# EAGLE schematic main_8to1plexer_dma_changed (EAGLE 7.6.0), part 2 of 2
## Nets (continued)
ZBUS0: IC6.3(1D) IC7.3(1D) IC48.3(1D) IC96.2(1A) IC97.2(1A) IC144.14(D1) IC175.4(B:I0) IC184.3(1D) IC189.3(1D) IC197.1(A:I0) IC216.3(1D) IC241.3(1C3) IC248.14(D1) RN5.1
ZBUS1: IC96.5(2A) IC97.5(2A) IC144.13(D2) IC175.5(B:I1) IC184.4(2D) IC197.2(A:I1) IC216.4(2D) IC243.3(1C3) IC248.13(D2) RN5.2
ZBUS2: IC96.11(3A) IC97.11(3A) IC144.12(D3) IC177.5(B:I1) IC184.7(3D) IC197.3(A:I2) IC216.7(3D) IC248.12(D3) IC255.3(1C3) RN5.3
ZBUS3: IC96.14(4A) IC97.14(4A) IC144.11(D4) IC184.8(4D) IC192.5(B:I1) IC197.12(A:I3) IC216.8(4D) IC248.11(D4) IC256.3(1C3) RN5.4
ZBUS4: IC94.2(1A) IC95.2(1A) IC128.14(D1) IC184.13(5D) IC193.5(B:I1) IC197.13(A:I4) IC208.3(1C3) IC216.13(5D) IC249.14(D1) RN5.5
ZBUS5: IC94.5(2A) IC95.5(2A) IC128.13(D2) IC184.14(6D) IC194.5(B:I1) IC199.2(A:I1) IC216.14(6D) IC249.13(D2) RN5.6
ZBUS6: IC94.11(3A) IC95.11(3A) IC128.12(D3) IC184.17(7D) IC199.3(A:I2) IC200.5(B:I1) IC216.17(7D) IC249.12(D3) RN5.7
ZBUS7: IC6.18(8D) IC7.18(8D) IC48.18(8D) IC80.5(B:I1) IC94.14(4A) IC95.14(4A) IC128.11(D4) IC184.18(8D) IC189.18(8D) IC199.12(A:I3) IC209.5(B:I1) IC216.18(8D) IC249.11(D4) IC255.5(1C1) RN5.8
ZF: IC120.2(A:I1) IC122.2(A1) IC155.6(1C0) IC227.2(Q1) IC241.6(1C0)
ZF_FROM_ALU: IC120.1(A:I0) IC121.2(1A) IC124.1(A:I0) IC127.1(A:I0) IC155.4(1C2) IC199.5(A:O) IC241.5(1C1)
ZF_IN_SRC_0: IC241.14(A)
ZF_IN_SRC_1: IC241.2(B)
~CLK: IC32.11(CLK) IC33.11(CLK)
~RST: IC32.1(CLR) IC33.1(CLR) IC44.4(A:PRE) IC54.4(B:O) IC162.1(CLR) IC195.1(A:I0) IC204.1(A:CLR) IC207.2(A:I1) IC218.1(A:I0) IC219.1(A:I0) IC220.2(A:I1) IC223.2(A:I1) IC224.2(A:I1) IC225.2(A:I1) IC227.1(CLR)
Unconnected: IC1.11(CLK) IC1.18(8D) IC2.12(Y7) IC2.13(Y6) IC2.14(Y5) IC3.12(Y7) IC3.13(Y6) IC3.14(Y5) IC4.11(CLK) IC5.11(CLK) IC6.4(2D) IC6.7(3D) IC6.8(4D) IC6.11(CLK) IC6.13(5D) IC6.14(6D) IC6.17(7D) IC7.4(2D) IC7.7(3D) IC7.8(4D) IC7.13(5D) IC7.14(6D) IC7.17(7D) IC8.6(A:!Q) IC8.8(B:!Q) IC8.9(B:Q) IC8.10(B:PRE) IC8.11(B:CLK) IC8.12(B:D) IC8.13(B:CLR) IC9.12(Y7) IC9.13(Y6) IC9.14(Y5) IC10.3(B:Y4) IC10.5(B:Y3) IC10.7(B:Y2) IC10.9(B:Y1) IC10.11(B:A1) IC10.13(B:A2) IC10.15(B:A3) IC10.17(B:A4) IC10.19(B:G) IC11.3(B:Y4) IC11.5(B:Y3) IC11.7(B:Y2) IC11.9(B:Y1) IC11.11(B:A1) IC11.13(B:A2) IC11.15(B:A3) IC11.17(B:A4) IC11.19(B:G) IC12.3(B:Y4) IC12.5(B:Y3) IC12.7(B:Y2) IC12.9(B:Y1) IC12.11(B:A1) IC12.13(B:A2) IC12.15(B:A3) IC12.17(B:A4) IC12.19(B:G) IC13.3(B:Y4) IC13.5(B:Y3) IC13.7(B:Y2) IC13.9(B:Y1) IC13.11(B:A1) IC13.13(B:A2) IC13.15(B:A3) IC13.17(B:A4) IC13.19(B:G) IC14.14(A=B) IC14.15(P) IC14.17(G) IC15.14(A=B) IC15.15(P) IC15.17(G) IC16.11(CLK) IC17.11(CLK) IC18.1(A:I0) IC18.2(A:I1) IC18.3(A:O) IC18.8(C:O) IC18.9(C:I0) IC18.10(C:I1) IC18.11(D:O) IC18.12(D:I0) IC18.13(D:I1) IC19.2(A1) IC19.3(A2) IC19.4(A3) IC19.5(A4) IC19.6(A5) IC19.7(A6) IC19.8(A7) IC19.9(A8) IC19.12(Y7) IC19.13(Y6) IC19.19(G2) IC20.1(D3) IC20.2(D2) IC20.3(D1) IC20.4(D0) IC20.6(W) IC20.7(G) IC20.9(C) IC20.10(B) IC20.11(A) IC20.12(D7) IC20.13(D6) IC20.14(D5) IC20.15(D4) IC21.11(CLK) IC24.1(A:G) IC24.2(A:A1) IC24.4(A:A2) IC24.6(A:A3) IC24.8(A:A4) IC24.12(A:Y4) IC24.14(A:Y3) IC24.16(A:Y2) IC24.18(A:Y1) IC25.1(A:G) IC25.2(A:A1) IC25.4(A:A2) IC25.6(A:A3) IC25.8(A:A4) IC25.12(A:Y4) IC25.14(A:Y3) IC25.16(A:Y2) IC25.18(A:Y1) IC26.1(A:G) IC26.2(A:A1) IC26.4(A:A2) IC26.6(A:A3) IC26.8(A:A4) IC26.12(A:Y4) IC26.14(A:Y3) IC26.16(A:Y2) IC26.18(A:Y1) IC27.1(A:G) IC27.2(A:A1) IC27.4(A:A2) IC27.6(A:A3) IC27.8(A:A4) IC27.12(A:Y4) IC27.14(A:Y3) IC27.16(A:Y2) IC27.18(A:Y1) IC28.12(Y7) IC28.13(Y6) IC28.14(Y5) IC29.12(Y7) IC29.13(Y6) IC29.14(Y5) IC30.3(B:Y4) IC30.5(B:Y3) IC30.7(B:Y2) IC30.9(B:Y1) IC30.11(B:A1) IC30.13(B:A2) IC30.15(B:A3) IC30.17(B:A4) IC30.19(B:G) IC31.3(B:Y4) IC31.5(B:Y3) IC31.7(B:Y2) IC31.9(B:Y1) IC31.11(B:A1) IC31.13(B:A2) IC31.15(B:A3) IC31.17(B:A4) IC31.19(B:G) IC34.6(W) IC34.7(G) IC34.9(C) IC34.10(B) IC34.11(A) IC34.12(D7) IC34.13(D6) IC35.6(W) IC35.7(G) IC35.9(C) IC35.10(B) IC35.11(A) IC35.12(D7) IC35.13(D6) IC36.6(W) IC36.7(G) IC36.9(C) IC36.10(B) IC36.11(A) IC36.12(D7) IC36.13(D6) IC37.6(W) IC37.7(G) IC37.9(C) IC37.10(B) IC37.11(A) IC37.12(D7) IC37.13(D6) IC38.6(W) IC38.7(G) IC38.9(C) IC38.10(B) IC38.11(A) IC38.12(D7) IC38.13(D6) IC39.4(B:I0) IC39.5(B:I1) IC39.6(B:O) IC39.8(C:O) IC39.9(C:I0) IC39.10(C:I1) IC39.11(D:O) IC39.12(D:I0) IC39.13(D:I1) IC40.6(W) IC40.7(G) IC40.9(C) IC40.10(B) IC40.11(A) IC40.12(D7) IC40.13(D6) IC41.6(W) IC41.7(G) IC41.9(C) IC41.10(B) IC41.11(A) IC41.12(D7) IC41.13(D6) IC42.4(B:I0) IC42.5(B:I1) IC42.6(B:O) IC42.8(C:O) IC42.9(C:I0) IC42.10(C:I1) IC42.11(D:O) IC42.12(D:I0) IC42.13(D:I1) IC43.1(A:I) IC43.2(A:O) IC43.5(C:I) IC43.6(C:O) IC43.8(D:O) IC43.9(D:I) IC43.10(E:O) IC43.11(E:I) IC43.12(F:O) IC43.13(F:I) IC44.6(A:!Q) IC44.8(B:!Q) IC44.9(B:Q) IC44.10(B:PRE) IC44.11(B:CLK) IC44.12(B:D) IC44.13(B:CLR) IC45.4(B:I0) IC45.5(B:I1) IC45.6(B:O) IC45.8(C:O) IC45.9(C:I0) IC45.10(C:I1) IC45.11(D:O) IC45.12(D:I0) IC45.13(D:I1) IC46.1(A:I0) IC46.2(A:I1) IC46.3(A:O) IC46.8(C:O) IC46.9(C:I0) IC46.10(C:I1) IC46.11(D:O) IC46.12(D:I0) IC46.13(D:I1) IC47.4(B:I0) IC47.5(B:I1) IC47.6(B:O) IC47.8(C:O) IC47.9(C:I0) IC47.10(C:I1) IC47.11(D:O) IC47.12(D:I0) IC47.13(D:I1) IC48.4(2D) IC48.7(3D) IC48.8(4D) IC48.11(CLK) IC48.13(5D) IC48.14(6D) IC48.17(7D) IC50.1(S2) IC50.10(S4) IC50.13(S3) IC51.1(S2) IC51.4(S1) IC51.10(S4) IC51.13(S3) IC52.1(S2) IC52.4(S1) IC52.10(S4) IC52.13(S3) IC53.4(S1) IC53.9(C4) IC53.10(S4) IC53.13(S3) IC54.1(A:I) IC54.2(A:O) IC54.5(C:I) IC54.6(C:O) IC54.8(D:O) IC54.9(D:I) IC54.10(E:O) IC54.11(E:I) IC54.12(F:O) IC54.13(F:I) IC56.9(2Y) IC56.10(2C0) IC56.11(2C1) IC56.12(2C2) IC56.13(2C3) IC57.5(C:I) IC57.6(C:O) IC57.8(D:O) IC57.9(D:I) IC57.10(E:O) IC57.11(E:I) IC57.12(F:O) IC57.13(F:I) IC58.4(B:I0) IC58.5(B:I1) IC58.6(B:O) IC58.8(C:O) IC58.9(C:I0) IC58.10(C:I1) IC58.11(D:O) IC58.12(D:I0) IC58.13(D:I1) IC59.3(B:I) IC59.4(B:O) IC59.5(C:I) IC59.6(C:O) IC59.8(D:O) IC59.9(D:I) IC59.10(E:O) IC59.11(E:I) IC59.12(F:O) IC59.13(F:I) IC60.1(CLR) IC60.9(Q4) IC60.12(Q5) IC60.15(Q6) IC60.16(Q7) IC60.19(Q8) IC61.1(CLR) IC61.2(Q1) IC61.5(Q2) IC61.6(Q3) IC61.9(Q4) IC61.12(Q5) IC61.15(Q6) IC61.16(Q7) IC61.19(Q8) IC62.1(CLR) IC62.2(Q1) IC62.5(Q2) IC62.6(Q3) IC62.9(Q4) IC62.12(Q5) IC62.15(Q6) IC62.16(Q7) IC62.19(Q8) IC64.3(B:I0) IC64.4(B:I1) IC64.5(B:I2) IC64.6(B:O) IC64.8(C:O) IC64.9(C:I0) IC64.10(C:I1) IC64.11(C:I2) IC65.4(B:O) IC65.5(B:I0) IC65.6(B:I1) IC65.8(C:I0) IC65.9(C:I1) IC65.10(C:O) IC65.11(D:I0) IC65.12(D:I1) IC65.13(D:O) IC66.4(B:O) IC66.5(B:I0) IC66.6(B:I1) IC66.8(C:I0) IC66.9(C:I1) IC66.10(C:O) IC66.11(D:I0) IC66.12(D:I1) IC66.13(D:O) IC67.1(A:I0) IC67.2(A:I1) IC67.3(A:O) IC67.8(C:O) IC67.9(C:I0) IC67.10(C:I1) IC67.11(D:O) IC67.12(D:I0) IC67.13(D:I1) IC68.9(3Y) IC68.12(4Y) IC69.1(A:G) IC69.2(A:A1) IC69.3(B:Y4) IC69.4(A:A2) IC69.6(A:A3) IC69.8(A:A4) IC69.12(A:Y4) IC69.14(A:Y3) IC69.16(A:Y2) IC69.18(A:Y1) IC70.6(W) IC71.6(W) IC71.7(G) IC71.9(C) IC71.10(B) IC71.11(A) IC71.12(D7) IC71.13(D6) IC72.1(A:I0) IC72.2(A:I1) IC72.3(A:O) IC72.8(C:O) IC72.9(C:I0) IC72.10(C:I1) IC72.11(D:O) IC72.12(D:I0) IC72.13(D:I1) IC73.6(W) IC73.7(G) IC73.9(C) IC73.10(B) IC73.11(A) IC73.12(D7) IC73.13(D6) IC74.1(A:I0) IC74.2(A:I1) IC74.3(A:O) IC74.8(C:O) IC74.9(C:I0) IC74.10(C:I1) IC74.11(D:O) IC74.12(D:I0) IC74.13(D:I1) IC75.2(Q1) IC75.5(Q2) IC75.6(Q3) IC75.9(Q4) IC75.12(Q5) IC75.15(Q6) IC75.16(Q7) IC75.19(Q8) IC76.2(Q1) IC77.2(Q1) IC78.2(Q1) IC78.5(Q2) IC78.6(Q3) IC78.9(Q4) IC78.12(Q5) IC78.15(Q6) IC78.16(Q7) IC78.19(Q8) IC79.2(Q1) IC79.5(Q2) IC79.6(Q3) IC79.9(Q4) IC79.12(Q5) IC79.15(Q6) IC79.16(Q7) IC79.19(Q8) IC80.1(A:I0) IC80.2(A:I1) IC80.3(A:O) IC80.8(C:O) IC80.9(C:I0) IC80.10(C:I1) IC80.11(D:O) IC80.12(D:I0) IC80.13(D:I1) IC81.1(A:I0) IC81.2(A:I1) IC81.3(A:O) IC81.8(C:O) IC81.9(C:I0) IC81.10(C:I1) IC81.11(D:O) IC81.12(D:I0) IC81.13(D:I1) IC82.11(CLK) IC83.1(A:I) IC83.2(A:O) IC83.5(C:I) IC83.6(C:O) IC83.8(D:O) IC83.9(D:I) IC83.10(E:O) IC83.11(E:I) IC83.12(F:O) IC83.13(F:I) IC84.1(A:I) IC84.2(A:O) IC84.5(C:I) IC84.6(C:O) IC84.8(D:O) IC84.9(D:I) IC84.10(E:O) IC84.11(E:I) IC84.12(F:O) IC84.13(F:I) IC85.3(B:I0) IC85.4(B:I1) IC85.5(B:I2) IC85.6(B:O) IC85.8(C:O) IC85.9(C:I0) IC85.10(C:I1) IC85.11(C:I2) IC86.11(CLK) IC87.2(A:S1) IC87.5(C:R) IC87.6(C:S) IC87.7(C:Q) IC87.9(B:Q) IC87.10(B:R) IC87.11(B:S1) IC87.12(B:S2) IC87.13(D:Q) IC87.14(D:R) IC87.15(D:S) IC88.11(CLK) IC89.3(B:Y4) IC89.5(B:Y3) IC89.7(B:Y2) IC89.9(B:Y1) IC89.11(B:A1) IC89.13(B:A2) IC89.15(B:A3) IC89.17(B:A4) IC89.19(B:G) IC90.3(B:Y4) IC90.5(B:Y3) IC90.7(B:Y2) IC90.9(B:Y1) IC90.11(B:A1) IC90.13(B:A2) IC90.15(B:A3) IC90.17(B:A4) IC90.19(B:G) IC91.3(B:Y4) IC91.5(B:Y3) IC91.7(B:Y2) IC91.9(B:Y1) IC91.11(B:A1) IC91.13(B:A2) IC91.15(B:A3) IC91.17(B:A4) IC91.19(B:G) IC92.3(B:Y4) IC92.5(B:Y3) IC92.7(B:Y2) IC92.9(B:Y1) IC92.11(B:A1) IC92.13(B:A2) IC92.15(B:A3) IC92.17(B:A4) IC92.19(B:G) IC93.11(CLK) IC98.11(CLK) IC99.11(CLK) IC100.11(CLK) IC101.11(CLK) IC102.12(Y7) IC102.13(Y6) IC102.14(Y5) IC103.12(Y7) IC103.13(Y6) IC103.14(Y5) IC103.15(Y4) IC103.16(Y3) IC103.17(Y2) IC104.12(Y7) IC104.13(Y6) IC104.14(Y5) IC104.15(Y4) IC104.16(Y3) IC104.17(Y2) IC105.1(A:G) IC105.2(A:A1) IC105.4(A:A2) IC105.6(A:A3) IC105.8(A:A4) IC105.12(A:Y4) IC105.14(A:Y3) IC105.16(A:Y2) IC105.18(A:Y1) IC106.1(A:G) IC106.2(A:A1) IC106.4(A:A2) IC106.6(A:A3) IC106.8(A:A4) IC106.12(A:Y4) IC106.14(A:Y3) IC106.16(A:Y2) IC106.18(A:Y1) IC107.1(A:G) IC107.2(A:A1) IC107.4(A:A2) IC107.6(A:A3) IC107.8(A:A4) IC107.12(A:Y4) IC107.14(A:Y3) IC107.16(A:Y2) IC107.18(A:Y1) IC108.1(A:G) IC108.2(A:A1) IC108.4(A:A2) IC108.6(A:A3) IC108.8(A:A4) IC108.12(A:Y4) IC108.14(A:Y3) IC108.16(A:Y2) IC108.18(A:Y1) IC109.1(A:G) IC109.2(A:A1) IC109.4(A:A2) IC109.6(A:A3) IC109.8(A:A4) IC109.12(A:Y4) IC109.14(A:Y3) IC109.16(A:Y2) IC109.18(A:Y1) IC110.1(A:G) IC110.2(A:A1) IC110.4(A:A2) IC110.6(A:A3) IC110.8(A:A4) IC110.12(A:Y4) IC110.14(A:Y3) IC110.16(A:Y2) IC110.18(A:Y1) IC111.1(A:G) IC111.2(A:A1) IC111.4(A:A2) IC111.6(A:A3) IC111.8(A:A4) IC111.12(A:Y4) IC111.14(A:Y3) IC111.16(A:Y2) IC111.18(A:Y1) IC112.1(A:G) IC112.2(A:A1) IC112.4(A:A2) IC112.6(A:A3) IC112.8(A:A4) IC112.12(A:Y4) IC112.14(A:Y3) IC112.16(A:Y2) IC112.18(A:Y1) IC113.13(Y6) IC113.14(Y5) IC113.19(G2) IC114.13(Y6) IC114.14(Y5) IC114.19(G2) IC115.13(Y6) IC115.14(Y5) IC117.12(Y7) IC117.13(Y6) IC117.14(Y5) IC118.6(3Q) IC118.7(3D) IC118.8(4D) IC118.9(4Q) IC118.11(CLK) IC118.12(5Q) IC118.13(5D) IC118.14(6D) IC118.15(6Q) IC118.16(7Q) IC118.17(7D) IC118.18(8D) IC118.19(8Q) IC119.1(A:I) IC119.2(A:O) IC119.5(C:I) IC119.6(C:O) IC119.8(D:O) IC119.9(D:I) IC119.10(E:O) IC119.11(E:I) IC119.12(F:O) IC119.13(F:I) IC120.4(B:I0) IC120.5(B:I1) IC120.6(B:O) IC120.8(C:O) IC120.9(C:I0) IC120.10(C:I1) IC120.11(D:O) IC120.12(D:I0) IC120.13(D:I1) IC121.4(1Y) IC121.5(2A) IC121.6(2B) IC121.7(2Y) IC121.9(3Y) IC121.10(3B) IC121.11(3A) IC121.12(4Y) IC121.13(4B) IC121.14(4A) IC122.12(Y7) IC122.13(Y6) IC122.14(Y5) IC123.11(CLK) IC123.18(8D) IC124.4(B:I0) IC124.5(B:I1) IC124.6(B:O) IC124.8(C:O) IC124.9(C:I0) IC124.10(C:I1) IC124.11(D:O) IC124.12(D:I0) IC124.13(D:I1) IC126.11(CLK) IC126.12(5Q) IC126.13(5D) IC126.14(6D) IC126.15(6Q) IC126.16(7Q) IC126.17(7D) IC126.18(8D) IC126.19(8Q) IC127.4(B:I0) IC127.5(B:I1) IC127.6(B:O) IC127.8(C:O) IC127.9(C:I0) IC127.10(C:I1) IC127.11(D:O) IC127.12(D:I0) IC127.13(D:I1) IC129.6(W) IC129.7(G) IC129.9(C) IC129.10(B) IC129.11(A) IC129.12(D7) IC129.13(D6) IC130.1(A:I0) IC130.2(A:I1) IC130.3(A:O) IC130.8(C:O) IC130.9(C:I0) IC130.10(C:I1) IC130.11(D:O) IC130.12(D:I0) IC130.13(D:I1) IC131.4(B:O) IC131.5(B:I0) IC131.6(B:I1) IC131.8(C:I0) IC131.9(C:I1) IC131.10(C:O) IC131.11(D:I0) IC131.12(D:I1) IC131.13(D:O) IC132.3(B:I0) IC132.4(B:I1) IC132.5(B:I2) IC132.6(B:O) IC132.8(C:O) IC132.9(C:I0) IC132.10(C:I1) IC132.11(C:I2) IC133.3(A:O) IC133.4(B:I0) IC133.5(B:I1) IC133.6(B:O) IC133.8(C:O) IC133.9(C:I0) IC133.10(C:I1) IC133.11(D:O) IC133.12(D:I0) IC133.13(D:I1) IC134.2(Q1) IC134.5(Q2) IC134.6(Q3) IC134.9(Q4) IC134.12(Q5) IC134.15(Q6) IC134.16(Q7) IC134.19(Q8) IC135.2(Q1) IC135.5(Q2) IC135.6(Q3) IC135.9(Q4) IC135.12(Q5) IC135.15(Q6) IC135.16(Q7) IC135.19(Q8) IC136.2(Q1) IC136.5(Q2) IC136.6(Q3) IC136.9(Q4) IC136.12(Q5) IC136.15(Q6) IC136.16(Q7) IC136.19(Q8) IC137.2(Q1) IC137.5(Q2) IC137.6(Q3) IC137.9(Q4) IC137.12(Q5) IC137.15(Q6) IC137.16(Q7) IC137.19(Q8) IC138.3(B:I0) IC138.4(B:I1) IC138.5(B:I2) IC138.6(B:O) IC138.8(C:O) IC138.9(C:I0) IC138.10(C:I1) IC138.11(C:I2) IC139.4(Q2) IC139.5(Q3) IC139.6(Q4) IC139.11(D4) IC139.12(D3) IC139.13(D2) IC140.12(Y7) IC140.13(Y6) IC140.14(Y5) IC140.15(Y4) IC140.16(Y3) IC140.17(Y2) IC141.3(B:I0) IC141.4(B:I1) IC141.5(B:I2) IC141.6(B:O) IC141.8(C:O) IC141.9(C:I0) IC141.10(C:I1) IC141.11(C:I2) IC142.6(W) IC142.7(G) IC142.9(C) IC142.10(B) IC142.11(A) IC142.12(D7) IC142.13(D6) IC143.4(B:I0) IC143.5(B:I1) IC143.6(B:O) IC143.8(C:O) IC143.9(C:I0) IC143.10(C:I1) IC143.11(D:O) IC143.12(D:I0) IC143.13(D:I1) IC145.12(Y7) IC145.13(Y6) IC145.14(Y5) IC146.12(Y7) IC146.13(Y6) IC146.14(Y5) IC147.1(A:I0) IC147.2(A:I1) IC147.3(A:O) IC147.8(C:O) IC147.9(C:I0) IC147.10(C:I1) IC147.11(D:O) IC147.12(D:I0) IC147.13(D:I1) IC148.4(B:I0) IC148.5(B:I1) IC148.6(B:O) IC148.8(C:O) IC148.9(C:I0) IC148.10(C:I1) IC148.11(D:O) IC148.12(D:I0) IC148.13(D:I1) IC149.1(A:I) IC149.2(A:O) IC149.5(C:I) IC149.6(C:O) IC149.8(D:O) IC149.9(D:I) IC149.10(E:O) IC149.11(E:I) IC149.12(F:O) IC149.13(F:I) IC150.3(B:I0) IC150.4(B:I1) IC150.5(B:I2) IC150.6(B:O) IC150.8(C:O) IC150.9(C:I0) IC150.10(C:I1) IC150.11(C:I2) IC151.3(B:I0) IC151.4(B:I1) IC151.5(B:I2) IC151.6(B:O) IC151.8(C:O) IC151.9(C:I0) IC151.10(C:I1) IC151.11(C:I2) IC152.1(A:I0) IC152.2(A:I1) IC152.3(A:O) IC152.4(B:I0) IC152.5(B:I1) IC152.6(B:O) IC152.11(D:O) IC152.12(D:I0) IC152.13(D:I1) IC153.11(CLK) IC155.3(1C3) IC155.13(2C3) IC156.3(1C3) IC156.13(2C3) IC157.3(B:I0) IC157.4(B:I1) IC157.5(B:I2) IC157.6(B:O) IC157.8(C:O) IC157.9(C:I0) IC157.10(C:I1) IC157.11(C:I2) IC158.3(B:I0) IC158.4(B:I1) IC158.5(B:I2) IC158.6(B:O) IC158.8(C:O) IC158.9(C:I0) IC158.10(C:I1) IC158.11(C:I2) IC159.6(W) IC159.7(G) IC159.9(C) IC159.10(B) IC159.11(A) IC159.12(D7) IC159.13(D6) IC160.6(W) IC160.7(G) IC160.9(C) IC160.10(B) IC160.11(A) IC160.12(D7) IC160.13(D6) IC161.4(B:I0) IC161.5(B:I1) IC161.6(B:O) IC161.8(C:O) IC161.9(C:I0) IC161.10(C:I1) IC161.11(D:O) IC161.12(D:I0) IC161.13(D:I1) IC163.6(A:!Q) IC163.8(B:!Q) IC163.9(B:Q) IC163.10(B:PRE) IC163.11(B:CLK) IC163.12(B:D) IC163.13(B:CLR) IC164.6(A:!Q) IC164.8(B:!Q) IC164.9(B:Q) IC164.10(B:PRE) IC164.11(B:CLK) IC164.12(B:D) IC164.13(B:CLR) IC165.11(CLK) IC166.11(CLK) IC167.5(2A) IC167.6(2B) IC167.7(2Y) IC167.9(3Y) IC167.10(3B) IC167.11(3A) IC167.12(4Y) IC167.13(4B) IC167.14(4A) IC168.6(A:!Q) IC168.8(B:!Q) IC168.9(B:Q) IC168.10(B:PRE) IC168.11(B:CLK) IC168.12(B:D) IC168.13(B:CLR) IC169.5(2Q) IC169.6(3Q) IC169.9(4Q) IC169.11(CLK) IC169.12(5Q) IC169.15(6Q) IC169.16(7Q) IC170.1(A:I0) IC170.2(A:I1) IC170.3(A:O) IC170.8(C:O) IC170.9(C:I0) IC170.10(C:I1) IC170.11(D:O) IC170.12(D:I0) IC170.13(D:I1) IC171.12(Y7) IC171.13(Y6) IC171.14(Y5) IC171.15(Y4) IC171.16(Y3) IC171.17(Y2) IC172.1(D3) IC172.2(D2) IC172.3(D1) IC172.4(D0) IC172.6(W) IC172.7(G) IC172.9(C) IC172.10(B) IC172.11(A) IC172.12(D7) IC172.13(D6) IC172.14(D5) IC172.15(D4) IC173.11(CLK) IC174.6(A:!Q) IC174.8(B:!Q) IC174.9(B:Q) IC174.10(B:PRE) IC174.11(B:CLK) IC174.12(B:D) IC174.13(B:CLR) IC175.1(A:I0) IC175.2(A:I1) IC175.3(A:O) IC175.8(C:O) IC175.9(C:I0) IC175.10(C:I1) IC175.11(D:O) IC175.12(D:I0) IC175.13(D:I1) IC176.3(B:Y4) IC176.5(B:Y3) IC176.7(B:Y2) IC176.9(B:Y1) IC176.11(B:A1) IC176.13(B:A2) IC176.15(B:A3) IC176.17(B:A4) IC176.19(B:G) IC177.1(A:I0) IC177.2(A:I1) IC177.3(A:O) IC177.8(C:O) IC177.9(C:I0) IC177.10(C:I1) IC177.11(D:O) IC177.12(D:I0) IC177.13(D:I1) IC178.3(B:Y4) IC178.5(B:Y3) IC178.7(B:Y2) IC178.9(B:Y1) IC178.11(B:A1) IC178.13(B:A2) IC178.15(B:A3) IC178.17(B:A4) IC178.19(B:G) IC179.3(B:Y4) IC179.5(B:Y3) IC179.7(B:Y2) IC179.9(B:Y1) IC179.11(B:A1) IC179.13(B:A2) IC179.15(B:A3) IC179.17(B:A4) IC179.19(B:G) IC180.11(CLK) IC181.3(B:Y4) IC181.5(B:Y3) IC181.7(B:Y2) IC181.9(B:Y1) IC181.11(B:A1) IC181.13(B:A2) IC181.15(B:A3) IC181.17(B:A4) IC181.19(B:G) IC182.3(B:Y4) IC182.5(B:Y3) IC182.7(B:Y2) IC182.9(B:Y1) IC182.11(B:A1) IC182.13(B:A2) IC182.15(B:A3) IC182.17(B:A4) IC182.19(B:G) IC183.3(B:Y4) IC183.5(B:Y3) IC183.7(B:Y2) IC183.9(B:Y1) IC183.11(B:A1) IC183.13(B:A2) IC183.15(B:A3) IC183.17(B:A4) IC183.19(B:G) IC184.11(CLK) IC185.11(CLK) IC186.6(W) IC186.7(G) IC186.9(C) IC186.10(B) IC186.11(A) IC186.12(D7) IC186.13(D6) IC187.6(A:!Q) IC187.8(B:!Q) IC187.9(B:Q) IC187.10(B:PRE) IC187.11(B:CLK) IC187.12(B:D) IC187.13(B:CLR) IC188.6(A:!Q) IC188.8(B:!Q) IC188.9(B:Q) IC188.10(B:PRE) IC188.11(B:CLK) IC188.12(B:D) IC188.13(B:CLR) IC189.4(2D) IC189.7(3D) IC189.8(4D) IC189.13(5D) IC189.14(6D) IC189.17(7D) IC190.1(A:I0) IC190.2(A:I1) IC190.3(A:O) IC190.4(B:I0) IC190.5(B:I1) IC190.6(B:O) IC190.11(D:O) IC190.12(D:I0) IC190.13(D:I1) IC191.3(B:I0) IC191.4(B:I1) IC191.5(B:I2) IC191.6(B:O) IC191.8(C:O) IC191.9(C:I0) IC191.10(C:I1) IC191.11(C:I2) IC192.1(A:I0) IC192.2(A:I1) IC192.3(A:O) IC192.8(C:O) IC192.9(C:I0) IC192.10(C:I1) IC192.11(D:O) IC192.12(D:I0) IC192.13(D:I1) IC193.1(A:I0) IC193.2(A:I1) IC193.3(A:O) IC193.8(C:O) IC193.9(C:I0) IC193.10(C:I1) IC193.11(D:O) IC193.12(D:I0) IC193.13(D:I1) IC194.1(A:I0) IC194.2(A:I1) IC194.3(A:O) IC194.8(C:O) IC194.9(C:I0) IC194.10(C:I1) IC194.11(D:O) IC194.12(D:I0) IC194.13(D:I1) IC195.4(B:I0) IC195.5(B:I1) IC195.6(B:O) IC195.8(C:O) IC195.9(C:I0) IC195.10(C:I1) IC195.11(D:O) IC195.12(D:I0) IC195.13(D:I1) IC196.1(A:I) IC196.2(A:O) IC196.5(C:I) IC196.6(C:O) IC196.8(D:O) IC196.9(D:I) IC196.10(E:O) IC196.11(E:I) IC196.12(F:O) IC196.13(F:I) IC197.4(B:I0) IC197.6(B:O) IC197.8(B:I1) IC197.9(B:I2) IC197.10(B:I3) IC197.11(B:I4) IC198.3(B:I) IC198.4(B:O) IC198.5(C:I) IC198.6(C:O) IC198.8(D:O) IC198.9(D:I) IC198.10(E:O) IC198.11(E:I) IC198.12(F:O) IC198.13(F:I) IC199.4(B:I0) IC199.6(B:O) IC199.8(B:I1) IC199.9(B:I2) IC199.10(B:I3) IC199.11(B:I4) IC200.1(A:I0) IC200.2(A:I1) IC200.3(A:O) IC200.8(C:O) IC200.9(C:I0) IC200.10(C:I1) IC200.11(D:O) IC200.12(D:I0) IC200.13(D:I1) IC201.1(A:I0) IC201.2(A:I1) IC201.3(A:O) IC201.4(B:I0) IC201.5(B:I1) IC201.6(B:O) IC201.11(D:O) IC201.12(D:I0) IC201.13(D:I1) IC202.4(B:I0) IC202.5(B:I1) IC202.6(B:O) IC202.8(C:O) IC202.9(C:I0) IC202.10(C:I1) IC202.11(D:O) IC202.12(D:I0) IC202.13(D:I1) IC203.1(A:I0) IC203.2(A:I1) IC203.3(A:O) IC203.4(B:I0) IC203.5(B:I1) IC203.6(B:O) IC203.11(D:O) IC203.12(D:I0) IC203.13(D:I1) IC204.6(A:!Q) IC204.8(B:!Q) IC204.9(B:Q) IC204.10(B:PRE) IC204.11(B:CLK) IC204.12(B:D) IC204.13(B:CLR) IC205.11(CLK) IC206.1(A:I0) IC206.2(A:I1) IC206.3(A:O) IC206.4(B:I0) IC206.5(B:I1) IC206.6(B:O) IC206.11(D:O) IC206.12(D:I0) IC206.13(D:I1) IC207.4(B:I0) IC207.5(B:I1) IC207.6(B:O) IC207.8(C:O) IC207.9(C:I0) IC207.10(C:I1) IC207.11(D:O) IC207.12(D:I0) IC207.13(D:I1) IC208.1(1G) IC208.9(2Y) IC208.10(2C0) IC208.11(2C1) IC208.12(2C2) IC208.13(2C3) IC208.15(2G) IC209.1(A:I0) IC209.2(A:I1) IC209.3(A:O) IC209.8(C:O) IC209.9(C:I0) IC209.10(C:I1) IC209.11(D:O) IC209.12(D:I0) IC209.13(D:I1) IC210.12(Y7) IC210.13(Y6) IC210.14(Y5) IC210.15(Y4) IC210.16(Y3) IC210.17(Y2) IC211.3(B:Y4) IC211.5(B:Y3) IC211.7(B:Y2) IC211.9(B:Y1) IC211.11(B:A1) IC211.13(B:A2) IC211.15(B:A3) IC211.17(B:A4) IC211.19(B:G) IC212.3(B:Y4) IC212.5(B:Y3) IC212.7(B:Y2) IC212.9(B:Y1) IC212.11(B:A1) IC212.13(B:A2) IC212.15(B:A3) IC212.17(B:A4) IC212.19(B:G) IC213.3(B:Y4) IC213.5(B:Y3) IC213.7(B:Y2) IC213.9(B:Y1) IC213.11(B:A1) IC213.13(B:A2) IC213.15(B:A3) IC213.17(B:A4) IC213.19(B:G) IC214.3(B:Y4) IC214.5(B:Y3) IC214.7(B:Y2) IC214.9(B:Y1) IC214.11(B:A1) IC214.13(B:A2) IC214.15(B:A3) IC214.17(B:A4) IC214.19(B:G) IC215.12(Y7) IC215.13(Y6) IC215.14(Y5) IC215.15(Y4) IC215.16(Y3) IC215.17(Y2) IC216.1(G) IC216.11(CLK) IC217.11(CLK) IC218.4(B:I0) IC218.5(B:I1) IC218.6(B:O) IC218.8(C:O) IC218.9(C:I0) IC218.10(C:I1) IC218.11(D:O) IC218.12(D:I0) IC218.13(D:I1) IC219.4(B:I0) IC219.5(B:I1) IC219.6(B:O) IC219.8(C:O) IC219.9(C:I0) IC219.10(C:I1) IC219.11(D:O) IC219.12(D:I0) IC219.13(D:I1) IC220.4(B:I0) IC220.5(B:I1) IC220.6(B:O) IC220.8(C:O) IC220.9(C:I0) IC220.10(C:I1) IC220.11(D:O) IC220.12(D:I0) IC220.13(D:I1) IC221.6(A:!Q) IC221.8(B:!Q) IC221.9(B:Q) IC221.10(B:PRE) IC221.11(B:CLK) IC221.12(B:D) IC221.13(B:CLR) IC223.4(B:I0) IC223.5(B:I1) IC223.6(B:O) IC223.8(C:O) IC223.9(C:I0) IC223.10(C:I1) IC223.11(D:O) IC223.12(D:I0) IC223.13(D:I1) IC224.4(B:I0) IC224.5(B:I1) IC224.6(B:O) IC224.8(C:O) IC224.9(C:I0) IC224.10(C:I1) IC224.11(D:O) IC224.12(D:I0) IC224.13(D:I1) IC225.4(B:I0) IC225.5(B:I1) IC225.6(B:O) IC225.8(C:O) IC225.9(C:I0) IC225.10(C:I1) IC225.11(D:O) IC225.12(D:I0) IC225.13(D:I1) IC227.11(CLK) IC228.1(A:I0) IC228.2(A:I1) IC228.3(A:O) IC228.4(B:I0) IC228.5(B:I1) IC228.6(B:O) IC228.11(D:O) IC228.12(D:I0) IC228.13(D:I1) IC229.3(B:Y4) IC229.5(B:Y3) IC229.7(B:Y2) IC229.9(B:Y1) IC229.11(B:A1) IC229.13(B:A2) IC229.15(B:A3) IC229.17(B:A4) IC229.19(B:G) IC230.3(B:Y4) IC230.5(B:Y3) IC230.7(B:Y2) IC230.9(B:Y1) IC230.11(B:A1) IC230.13(B:A2) IC230.15(B:A3) IC230.17(B:A4) IC230.19(B:G) IC231.3(B:Y4) IC231.5(B:Y3) IC231.7(B:Y2) IC231.9(B:Y1) IC231.11(B:A1) IC231.13(B:A2) IC231.15(B:A3) IC231.17(B:A4) IC231.19(B:G) IC232.3(B:Y4) IC232.5(B:Y3) IC232.7(B:Y2) IC232.9(B:Y1) IC232.11(B:A1) IC232.13(B:A2) IC232.15(B:A3) IC232.17(B:A4) IC232.19(B:G) IC233.11(CLK) IC234.11(CLK) IC235.3(B:Y4) IC235.5(B:Y3) IC235.7(B:Y2) IC235.9(B:Y1) IC235.11(B:A1) IC235.13(B:A2) IC235.15(B:A3) IC235.17(B:A4) IC235.19(B:G) IC236.3(B:Y4) IC236.5(B:Y3) IC236.7(B:Y2) IC236.9(B:Y1) IC236.11(B:A1) IC236.13(B:A2) IC236.15(B:A3) IC236.17(B:A4) IC236.19(B:G) IC237.3(B:Y4) IC237.5(B:Y3) IC237.7(B:Y2) IC237.9(B:Y1) IC237.11(B:A1) IC237.13(B:A2) IC237.15(B:A3) IC237.17(B:A4) IC237.19(B:G) IC238.3(B:Y4) IC238.5(B:Y3) IC238.7(B:Y2) IC238.9(B:Y1) IC238.11(B:A1) IC238.13(B:A2) IC238.15(B:A3) IC238.17(B:A4) IC238.19(B:G) IC239.11(CLK) IC240.11(CLK) IC241.1(1G) IC241.9(2Y) IC241.10(2C0) IC241.11(2C1) IC241.12(2C2) IC241.13(2C3) IC241.15(2G) IC242.1(A:I0) IC242.2(A:I1) IC242.3(A:O) IC242.4(B:I0) IC242.5(B:I1) IC242.6(B:O) IC242.11(D:O) IC242.12(D:I0) IC242.13(D:I1) IC243.1(1G) IC243.9(2Y) IC243.10(2C0) IC243.11(2C1) IC243.12(2C2) IC243.13(2C3) IC243.15(2G) IC244.1(A:G) IC244.2(A:A1) IC244.4(A:A2) IC244.5(B:Y3) IC244.6(A:A3) IC244.7(B:Y2) IC244.8(A:A4) IC244.12(A:Y4) IC244.14(A:Y3) IC244.16(A:Y2) IC244.18(A:Y1) IC246.11(CLK) IC247.1(A:G) IC247.2(A:A1) IC247.4(A:A2) IC247.5(B:Y3) IC247.6(A:A3) IC247.7(B:Y2) IC247.8(A:A4) IC247.12(A:Y4) IC247.14(A:Y3) IC247.16(A:Y2) IC247.18(A:Y1) IC250.1(A:I0) IC250.2(A:I1) IC250.3(A:O) IC250.8(C:O) IC250.9(C:I0) IC250.10(C:I1) IC250.11(D:O) IC250.12(D:I0) IC250.13(D:I1) IC255.1(1G) IC255.9(2Y) IC255.10(2C0) IC255.11(2C1) IC255.12(2C2) IC255.13(2C3) IC255.15(2G) IC256.1(1G) IC256.9(2Y) IC256.10(2C0) IC256.11(2C1) IC256.12(2C2) IC256.13(2C3) IC256.15(2G) IC257.15(G) IC259.12(Y7) IC259.13(Y6) IC259.14(Y5) IC259.15(Y4) IC259.16(Y3) IC259.17(Y2) IC260.12(Y7) IC260.13(Y6) IC260.14(Y5) IC260.15(Y4) IC260.16(Y3) IC260.17(Y2) IC261.11(CLK) IC262.11(CLK) IC263.12(Y7) IC263.13(Y6) IC263.14(Y5) IC263.15(Y4) IC263.16(Y3) IC263.17(Y2) IC264.12(Y7) IC264.13(Y6) IC264.14(Y5) IC264.15(Y4) IC264.16(Y3) IC264.17(Y2) RN4.4 RN4.5 RN4.6 RN4.7 RN4.8 RN4.9 RN4.10 RN4.11 RN4.12 RN4.13 S2.1(O) S4.1(O) SW3.8 U$1.28(VCC) U$2.28(VCC) U$3.28(VCC) U$4.28(VCC) U$5.28(VCC) U$6.28(VCC) U$7.28(VCC) U$8.28(VCC) U$9.28(VCC) U$10.1(A14) U$10.2(A12) U$10.3(A7) U$10.4(A6) U$10.5(A5) U$10.6(A4) U$10.7(A3) U$10.8(A2) U$10.9(A1) U$10.10(A0) U$10.14(GND) U$10.20(/CE) U$10.21(A10) U$10.22(/OE) U$10.23(A11) U$10.24(A9) U$10.25(A8) U$10.26(A13) U$10.27(/WE) U$10.28(VCC) U$11.1(A14) U$11.2(A12) U$11.3(A7) U$11.4(A6) U$11.5(A5) U$11.6(A4) U$11.7(A3) U$11.8(A2) U$11.9(A1) U$11.10(A0) U$11.14(GND) U$11.20(/CE) U$11.21(A10) U$11.22(/OE) U$11.23(A11) U$11.24(A9) U$11.25(A8) U$11.26(A13) U$11.27(/WE) U$11.28(VCC) U$12.1(A14) U$12.2(A12) U$12.3(A7) U$12.4(A6) U$12.5(A5) U$12.6(A4) U$12.7(A3) U$12.8(A2) U$12.9(A1) U$12.10(A0) U$12.14(GND) U$12.20(/CE) U$12.21(A10) U$12.22(/OE) U$12.23(A11) U$12.24(A9) U$12.25(A8) U$12.26(A13) U$12.27(/WE) U$12.28(VCC)

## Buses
XBUS[0..7]
ZBUS[0..7]
YBUS[0..7]
AD[0..15]
MDR_IN_BUS[0..7]
U_AD[0..15]
DATA[0..7]

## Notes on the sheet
- SYNCHRONIZED INTERRUPT INPUTS
- TRAP
  INT_REQ_0
  INT_REQ_1
  INT_REQ_2
  INT_REQ_3
  INT_REQ_4
  INT_REQ_5
  INT_REQ_6
- R_SHIFT_L
- SINGLE STEP CLOCK
- might need to flip flop this output in case it oscillates
- fast clock
- slow clock
- R_SHIFT_H
- the encoded bits start at position 3 in the byte. 
  this is so it's easier to just transfer this to PC and 
  have it become the interrupt vector in memory.
  
  so each interrupt spans 8 bytes in memory.
  
  00000000 = int_0
  00001000 = int_1
  00010000 = int_2
  00011000 = int_3
  etc
- IMMX
- TDR0_L
- TDR0_H
- TDR1_L
- U-ADDRESS MUX
- TDR1_H
- CS_L
- CS_H
- MASK_FLAGS
- DS_L
- OFFSET(6)
- IR_L
- DS_H
- AL
- Z BUS
- PC_L
- U-CODE ROMS
- U-ADDRESS
- U-CODE FF'S
- SS_L
- IR_H
- AH
- ADDRESS & DATA BUSES NEED PULL DOWN RESISTORS 
  BECAUSE THE CPU BUS OUTPUTS HAVE 
  244'S WHICH ARE CLOSED MOST OF THE TIME.
- LOW | ADDRESS BUS | PC_H
- MARL
- SS_H
- LOW
- ADDER
- BL
- HIGH
- SP_L
- ES_L
- BH
- ADDER
- MARH
- MAR is tri-stated when in programming or DMA mode. | SP_H
- ES_H
- programming mode signal goes here to tell MAR to go tristate
- AUX_FLAGS
- CL
- BP_L
- CH
- if type = branch, and condition = false, then next = +1
- HIGH
- BP_H
- DL
- Z BUS
- FLAGS REGISTER
- DH
- CARRY IN MUX
- U_FLAGS
- BUS GOING INTO MDR INPUTS
- X BUS
- DATA BUS
- CONDITION SOURCE
  PROGRAMMER'S FLAGS 
  OR
  U_CODE FLAGS
- MDR_L
- ZF
- CF / LTU
- MDR_H
- SF | MDR MUX | BUS GOING INTO MDR INPUTS
- IMMY
- OF
- PF
- ALU
- LT
  LTE
  ~LT = GTE
  ~LTE + GT
- alu_mode removed. OF is undefined if alu in logic mode anyway. | alu_op == add
- DATA BUS
- SERIES TERMINATION ~80 ohm
- ALU_OP == SUB
- TDR0_L
- IMMY
- TDR0_H
- FROM MICROCODE
- TDR1_L
- TDR1_H
- THESE TDR'S ARE THE SAME ONES AS ARE CONNECTED TO THE X BUS

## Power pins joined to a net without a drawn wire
GND: IC1.10(GND) IC2.10(GND) IC3.10(GND) IC4.10(GND) IC5.10(GND) IC6.10(GND) IC7.10(GND) IC8.7(P:GND) IC9.10(GND) IC10.10(P:GND) IC11.10(P:GND) IC12.10(P:GND) IC13.10(P:GND) IC14.12(GND) IC15.12(GND) IC16.10(GND) IC17.10(GND) IC18.7(P:GND) IC19.10(GND) IC20.8(GND) IC21.10(GND) IC22.8(GND) IC23.8(GND) IC24.10(P:GND) IC25.10(P:GND) IC26.10(P:GND) IC27.10(P:GND) IC28.10(GND) IC29.10(GND) IC30.10(P:GND) IC31.10(P:GND) IC32.10(GND) IC33.10(GND) IC34.8(GND) IC35.8(GND) IC36.8(GND) IC37.8(GND) IC38.8(GND) IC39.7(P:GND) IC40.8(GND) IC41.8(GND) IC42.7(P:GND) IC43.7(P:GND) IC44.7(P:GND) IC45.7(P:GND) IC46.7(P:GND) IC47.7(P:GND) IC48.10(GND) IC49.8(GND) IC50.8(GND) IC51.8(GND) IC52.8(GND) IC53.8(GND) IC54.7(P:GND) IC55.8(GND) IC56.8(GND) IC57.7(P:GND) IC58.7(P:GND) IC59.7(P:GND) IC60.10(GND) IC61.10(GND) IC62.10(GND) IC63.8(GND) IC64.7(P:GND) IC65.7(P:GND) IC66.7(P:GND) IC67.7(P:GND) IC68.8(GND) IC69.10(P:GND) IC70.8(GND) IC71.8(GND) IC72.7(P:GND) IC73.8(GND) IC74.7(P:GND) IC75.10(GND) IC76.10(GND) IC77.10(GND) IC78.10(GND) IC79.10(GND) IC80.7(P:GND) IC81.7(P:GND) IC82.10(GND) IC83.7(P:GND) IC84.7(P:GND) IC85.7(P:GND) IC86.10(GND) IC87.8(P:GND) IC88.10(GND) IC89.10(P:GND) IC90.10(P:GND) IC91.10(P:GND) IC92.10(P:GND) IC93.10(GND) IC94.8(GND) IC95.8(GND) IC96.8(GND) IC97.8(GND) IC98.10(GND) IC99.10(GND) IC100.10(GND) IC101.10(GND) IC102.10(GND) IC103.10(GND) IC104.10(GND) IC105.10(P:GND) IC106.10(P:GND) IC107.10(P:GND) IC108.10(P:GND) IC109.10(P:GND) IC110.10(P:GND) IC111.10(P:GND) IC112.10(P:GND) IC113.10(GND) IC114.10(GND) IC115.10(GND) IC116.10(GND) IC117.10(GND) IC118.10(GND) IC119.7(P:GND) IC120.7(P:GND) IC121.8(GND) IC122.10(GND) IC123.10(GND) IC124.7(P:GND) IC125.10(GND) IC126.10(GND) IC127.7(P:GND) IC128.8(GND) IC129.8(GND) IC130.7(P:GND) IC131.7(P:GND) IC132.7(P:GND) IC133.7(P:GND) IC134.10(GND) IC135.10(GND) IC136.10(GND) IC137.10(GND) IC138.7(P:GND) IC139.8(GND) IC140.10(GND) IC141.7(P:GND) IC142.8(GND) IC143.7(P:GND) IC144.8(GND) IC145.10(GND) IC146.10(GND) IC147.7(P:GND) IC148.7(P:GND) IC149.7(P:GND) IC150.7(P:GND) IC151.7(P:GND) IC152.7(P:GND) IC153.10(GND) IC154.10(GND) IC155.8(GND) IC156.8(GND) IC157.7(P:GND) IC158.7(P:GND) IC159.8(GND) IC160.8(GND) IC161.7(P:GND) IC162.10(GND) IC163.7(P:GND) IC164.7(P:GND) IC165.10(GND) IC166.10(GND) IC167.8(GND) IC168.7(P:GND) IC169.10(GND) IC170.7(P:GND) IC171.10(GND) IC172.8(GND) IC173.10(GND) IC174.7(P:GND) IC175.7(P:GND) IC176.10(P:GND) IC177.7(P:GND) IC178.10(P:GND) IC179.10(P:GND) IC180.10(GND) IC181.10(P:GND) IC182.10(P:GND) IC183.10(P:GND) IC184.10(GND) IC185.10(GND) IC186.8(GND) IC187.7(P:GND) IC188.7(P:GND) IC189.10(GND) IC190.7(P:GND) IC191.7(P:GND) IC192.7(P:GND) IC193.7(P:GND) IC194.7(P:GND) IC195.7(P:GND) IC196.7(P:GND) IC197.7(P:GND) IC198.7(P:GND) IC199.7(P:GND) IC200.7(P:GND) IC201.7(P:GND) IC202.7(P:GND) IC203.7(P:GND) IC204.7(P:GND) IC205.10(GND) IC206.7(P:GND) IC207.7(P:GND) IC208.8(GND) IC209.7(P:GND) IC210.10(GND) IC211.10(P:GND) IC212.10(P:GND) IC213.10(P:GND) IC214.10(P:GND) IC215.10(GND) IC216.10(GND) IC217.10(GND) IC218.7(P:GND) IC219.7(P:GND) IC220.7(P:GND) IC221.7(P:GND) IC222.8(GND) IC223.7(P:GND) IC224.7(P:GND) IC225.7(P:GND) IC226.8(GND) IC227.10(GND) IC228.7(P:GND) IC229.10(P:GND) IC230.10(P:GND) IC231.10(P:GND) IC232.10(P:GND) IC233.10(GND) IC234.10(GND) IC235.10(P:GND) IC236.10(P:GND) IC237.10(P:GND) IC238.10(P:GND) IC239.10(GND) IC240.10(GND) IC241.8(GND) IC242.7(P:GND) IC243.8(GND) IC244.10(P:GND) IC245.10(GND) IC246.10(GND) IC247.10(P:GND) IC248.8(GND) IC249.8(GND) IC250.7(P:GND) IC255.8(GND) IC256.8(GND) IC257.8(GND) IC258.8(GND) IC259.10(GND) IC260.10(GND) IC261.10(GND) IC262.10(GND) IC263.10(GND) IC264.10(GND)
VCC: IC1.20(VCC) IC2.20(VCC) IC3.20(VCC) IC4.20(VCC) IC5.20(VCC) IC6.20(VCC) IC7.20(VCC) IC8.14(P:VCC) IC9.20(VCC) IC10.20(P:VCC) IC11.20(P:VCC) IC12.20(P:VCC) IC13.20(P:VCC) IC14.24(VCC) IC15.24(VCC) IC16.20(VCC) IC17.20(VCC) IC18.14(P:VCC) IC19.20(VCC) IC20.16(VCC) IC21.20(VCC) IC22.16(VCC) IC23.16(VCC) IC24.20(P:VCC) IC25.20(P:VCC) IC26.20(P:VCC) IC27.20(P:VCC) IC28.20(VCC) IC29.20(VCC) IC30.20(P:VCC) IC31.20(P:VCC) IC32.20(VCC) IC33.20(VCC) IC34.16(VCC) IC35.16(VCC) IC36.16(VCC) IC37.16(VCC) IC38.16(VCC) IC39.14(P:VCC) IC40.16(VCC) IC41.16(VCC) IC42.14(P:VCC) IC43.14(P:VCC) IC44.14(P:VCC) IC45.14(P:VCC) IC46.14(P:VCC) IC47.14(P:VCC) IC48.20(VCC) IC49.16(VCC) IC50.16(VCC) IC51.16(VCC) IC52.16(VCC) IC53.16(VCC) IC54.14(P:VCC) IC55.16(VCC) IC56.16(VCC) IC57.14(P:VCC) IC58.14(P:VCC) IC59.14(P:VCC) IC60.20(VCC) IC61.20(VCC) IC62.20(VCC) IC63.16(VCC) IC64.14(P:VCC) IC65.14(P:VCC) IC66.14(P:VCC) IC67.14(P:VCC) IC68.16(VCC) IC69.20(P:VCC) IC70.16(VCC) IC71.16(VCC) IC72.14(P:VCC) IC73.16(VCC) IC74.14(P:VCC) IC75.20(VCC) IC76.20(VCC) IC77.20(VCC) IC78.20(VCC) IC79.20(VCC) IC80.14(P:VCC) IC81.14(P:VCC) IC82.20(VCC) IC83.14(P:VCC) IC84.14(P:VCC) IC85.14(P:VCC) IC86.20(VCC) IC87.16(P:VCC) IC88.20(VCC) IC89.20(P:VCC) IC90.20(P:VCC) IC91.20(P:VCC) IC92.20(P:VCC) IC93.20(VCC) IC94.16(VCC) IC95.16(VCC) IC96.16(VCC) IC97.16(VCC) IC98.20(VCC) IC99.20(VCC) IC100.20(VCC) IC101.20(VCC) IC102.20(VCC) IC103.20(VCC) IC104.20(VCC) IC105.20(P:VCC) IC106.20(P:VCC) IC107.20(P:VCC) IC108.20(P:VCC) IC109.20(P:VCC) IC110.20(P:VCC) IC111.20(P:VCC) IC112.20(P:VCC) IC113.20(VCC) IC114.20(VCC) IC115.20(VCC) IC116.20(VCC) IC117.20(VCC) IC118.20(VCC) IC119.14(P:VCC) IC120.14(P:VCC) IC121.16(VCC) IC122.20(VCC) IC123.20(VCC) IC124.14(P:VCC) IC125.20(VCC) IC126.20(VCC) IC127.14(P:VCC) IC128.16(VCC) IC129.16(VCC) IC130.14(P:VCC) IC131.14(P:VCC) IC132.14(P:VCC) IC133.14(P:VCC) IC134.20(VCC) IC135.20(VCC) IC136.20(VCC) IC137.20(VCC) IC138.14(P:VCC) IC139.16(VCC) IC140.20(VCC) IC141.14(P:VCC) IC142.16(VCC) IC143.14(P:VCC) IC144.16(VCC) IC145.20(VCC) IC146.20(VCC) IC147.14(P:VCC) IC148.14(P:VCC) IC149.14(P:VCC) IC150.14(P:VCC) IC151.14(P:VCC) IC152.14(P:VCC) IC153.20(VCC) IC154.20(VCC) IC155.16(VCC) IC156.16(VCC) IC157.14(P:VCC) IC158.14(P:VCC) IC159.16(VCC) IC160.16(VCC) IC161.14(P:VCC) IC162.20(VCC) IC163.14(P:VCC) IC164.14(P:VCC) IC165.20(VCC) IC166.20(VCC) IC167.16(VCC) IC168.14(P:VCC) IC169.20(VCC) IC170.14(P:VCC) IC171.20(VCC) IC172.16(VCC) IC173.20(VCC) IC174.14(P:VCC) IC175.14(P:VCC) IC176.20(P:VCC) IC177.14(P:VCC) IC178.20(P:VCC) IC179.20(P:VCC) IC180.20(VCC) IC181.20(P:VCC) IC182.20(P:VCC) IC183.20(P:VCC) IC184.20(VCC) IC185.20(VCC) IC186.16(VCC) IC187.14(P:VCC) IC188.14(P:VCC) IC189.20(VCC) IC190.14(P:VCC) IC191.14(P:VCC) IC192.14(P:VCC) IC193.14(P:VCC) IC194.14(P:VCC) IC195.14(P:VCC) IC196.14(P:VCC) IC197.14(P:VCC) IC198.14(P:VCC) IC199.14(P:VCC) IC200.14(P:VCC) IC201.14(P:VCC) IC202.14(P:VCC) IC203.14(P:VCC) IC204.14(P:VCC) IC205.20(VCC) IC206.14(P:VCC) IC207.14(P:VCC) IC208.16(VCC) IC209.14(P:VCC) IC210.20(VCC) IC211.20(P:VCC) IC212.20(P:VCC) IC213.20(P:VCC) IC214.20(P:VCC) IC215.20(VCC) IC216.20(VCC) IC217.20(VCC) IC218.14(P:VCC) IC219.14(P:VCC) IC220.14(P:VCC) IC221.14(P:VCC) IC222.16(VCC) IC223.14(P:VCC) IC224.14(P:VCC) IC225.14(P:VCC) IC226.16(VCC) IC227.20(VCC) IC228.14(P:VCC) IC229.20(P:VCC) IC230.20(P:VCC) IC231.20(P:VCC) IC232.20(P:VCC) IC233.20(VCC) IC234.20(VCC) IC235.20(P:VCC) IC236.20(P:VCC) IC237.20(P:VCC) IC238.20(P:VCC) IC239.20(VCC) IC240.20(VCC) IC241.16(VCC) IC242.14(P:VCC) IC243.16(VCC) IC244.20(P:VCC) IC245.20(VCC) IC246.20(VCC) IC247.20(P:VCC) IC248.16(VCC) IC249.16(VCC) IC250.14(P:VCC) IC255.16(VCC) IC256.16(VCC) IC257.16(VCC) IC258.16(VCC) IC259.20(VCC) IC260.20(VCC) IC261.20(VCC) IC262.20(VCC) IC263.20(VCC) IC264.20(VCC)

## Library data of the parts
IC1 IC4-IC7 IC16 IC17 IC21 IC48 IC82 IC86 IC88 IC93 IC98-IC101 IC118 IC123 IC153 IC165 IC166 IC169 IC173 IC180 IC184 IC185 IC189 IC205 IC216 IC217 IC233 IC234 IC239 IC240 IC246 IC261 IC262 = 74xx-us:74*377: Octal D type FLIP FLOP, enable
IC2 IC3 IC9 IC19 IC28 IC29 IC102-IC104 IC113-IC117 IC122 IC125 IC140 IC145 IC146 IC154 IC171 IC210 IC215 IC245 IC259 IC260 IC263 IC264 = 74xx-us:74*541: Octal BUFFER and LINE DRIVER, 3-state; OC_FARNELL: unknown
IC8 IC163 IC164 IC168 IC174 IC187 IC188 IC204 IC221 = 74xx-us:74*74: Dual D type positive edge triggered FLIP FLOP, preset and clear
IC10-IC13 IC24-IC27 IC30 IC31 IC69 IC105-IC112 IC176 IC178 IC179 IC181-IC183 IC244 IC247 = 74xx-us:74*244: Octal BUFFER and LINE DRIVER, 3-state; MF: TEXAS INSTRUMENTS; MPN: SN74LS244N; OC_FARNELL: 1739688
IC14 IC15 = 74xx-us:74*181: ARITHMETIC LOGIC UNIT function generator; OC_FARNELL: unknown
IC18 IC46 IC67 IC81 IC147 IC170 IC250 = 74xx-us:74*32: Quad 2-input OR gate; MF: TEXAS INSTRUMENTS; MPN: SN7432N; OC_FARNELL: 1607803
IC20 IC34-IC38 IC40 IC41 IC70 IC71 IC73 IC129 IC142 IC159 IC160 IC172 IC186 = 74xx-us:74*151: Data SELECTOR/MULTIPLEXER
IC22 IC23 IC94-IC97 IC121 IC167 IC257 IC258 = 74xx-us:74*157: Quadruple 2-line to 1-line data SELECTOR/MULTIPLEXER; OC_FARNELL: unknown
IC32 IC33 IC60-IC62 IC75-IC79 IC134-IC137 = 74xx-us:74*273: Octal D type FLIP FLOP, clear; OC_FARNELL: unknown
IC39 IC42 IC45 IC47 IC120 IC124 IC127 IC133 IC143 IC148 IC161 IC195 IC202 IC207 IC218-IC220 IC223-IC225 = 74xx-us:74*08: Quad 2-input AND gate; OC_FARNELL: unknown
IC43 IC54 IC57 IC59 IC83 IC84 IC119 IC198 = 74xx-us:74*04: Hex INVERTER; OC_FARNELL: unknown
IC44 = 74xx-us:74*74: Dual D type positive edge triggered FLIP FLOP, preset and clear; OC_FARNELL: unknown
IC49 IC55 IC63 IC68 = 74xx-us:74*257: Quadruple 2-to 1 line data SELECTOR/MULTIPLEXER; OC_FARNELL: unknown
IC50-IC53 = 74xx-us:74*283: 4-bit binary FULL ADDER, fast carry; OC_FARNELL: unknown
IC56 IC155 IC156 IC208 IC241 IC243 IC255 IC256 = 74xx-us:74*153: Dual 4-line to 1-line data SELECTOR/MULTIPLEXER; OC_FARNELL: unknown
IC58 IC72 IC74 IC80 IC130 IC175 IC177 IC192-IC194 IC200 IC209 = 74xx-us:74*86: Quad 2-input EXCLUSIV-OR (XOR) gate; OC_FARNELL: unknown
IC64 IC85 IC132 IC138 IC150 IC151 IC157 IC158 IC191 = 74xx-us:74*10: Triple 3-input NAND gate
IC65 IC66 IC131 = 74xx-us:74*02: Quad 2-input NOR gate
IC87 = 74xx-us:74*279: Quadruple S-R LATCH; OC_FARNELL: unknown
IC89-IC92 IC211-IC214 IC229-IC232 IC235-IC238 = 74xx-us:74*244: Octal BUFFER and LINE DRIVER, 3-state; OC_FARNELL: unknown
IC126 = 74xx-us:74*377: Octal D type FLIP FLOP, enable; OC_FARNELL: unknown
IC128 IC144 IC248 IC249 = 74xx-us:74*173: 4-bit D type REGISTER, 3-state
IC139 = 74xx-us:74*173: 4-bit D type REGISTER, 3-state; OC_FARNELL: unknown
IC141 = 74xx-us:74*11: Triple 3-input AND gate
IC149 IC196 = 74xx-us:74*04: Hex INVERTER
IC152 IC190 IC201 IC203 IC206 IC228 IC242 = 74xx-us:74*00: Quad 2-input NAND gate
IC162 IC227 = 74xx-us:74*273: Octal D type FLIP FLOP, clear
IC197 IC199 = 74xx-us:74*260: Dual 5-input positive NOR gate; OC_FARNELL: unknown
IC222 = 74xx-us:74*138: 3-line to 8-line DECODER/DEMULTIPLEXER
IC226 = 74xx-us:74*148: 10-line to 4-line and 8-line to 3-line PRIORITY ENCODER
R1-R3 R9 = rcl:R-US_: RESISTOR, American symbol; OC_FARNELL: unknown
R5-R8 R10-R14 = resistor:R-US_: RESISTOR, American symbol
RN1-RN5 = resistor-dil:8R-N: DIL RESISTOR; OC_FARNELL: unknown; OC_NEWARK: unknown
S1 S2 S4 = switch:TL36PO: TINY SWITCH ON - ON Source: http://www2.produktinfo.conrad.com/datenblaetter/700000-724999/705152-da-01-de-Subminiaturschalter_TL_36YO.pdf; OC_FARNELL: unknown
SW3 = special:SW-C10: SWITCH 10-step rotary switch; OC_FARNELL: unknown
U$1-U$12 = atmel_28c:AT28C256-28DIP: IC EEPROM 256KBIT 150NS 28DIP; OC_FARNELL: unknown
